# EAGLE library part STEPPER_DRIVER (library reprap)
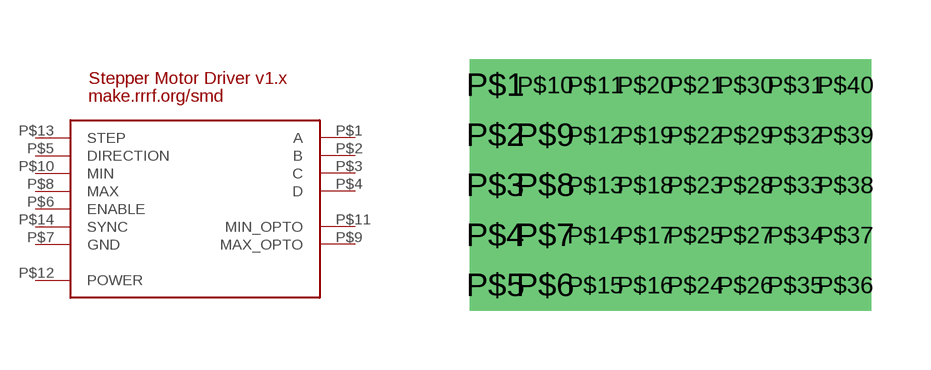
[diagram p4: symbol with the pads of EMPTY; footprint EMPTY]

Designator prefix -

## STEPPER_DRIVER  [EMPTY]
P$1  A
P$2  B
P$3  C
P$4  D
P$5  DIRECTION
P$6  ENABLE
P$7  GND
P$8  MAX
P$9  MAX_OPTO
P$10  MIN
P$11  MIN_OPTO
P$12  POWER
P$13  STEP
P$14  SYNC

## Footprint EMPTY (pad centres in mm)
drill 0.8 square: P$1 -1.27,5.08; P$2 -1.27,3.81; P$3 -1.27,2.54; P$4 -1.27,1.27; P$5 -1.27,0; P$6 0,0; P$7 0,1.27; P$8 0,2.54; P$9 0,3.81; P$10 0,5.08; P$11 1.27,5.08; P$12 1.27,3.81; P$13 1.27,2.54; P$14 1.27,1.27; P$15 1.27,0; P$16 2.54,0; P$17 2.54,1.27; P$18 2.54,2.54; P$19 2.54,3.81; P$20 2.54,5.08; P$21 3.81,5.08; P$22 3.81,3.81; P$23 3.81,2.54; P$24 3.81,0; P$25 3.81,1.27; P$26 5.08,0; P$27 5.08,1.27; P$28 5.08,2.54; P$29 5.08,3.81; P$30 5.08,5.08; P$31 6.35,5.08; P$32 6.35,3.81; P$33 6.35,2.54; P$34 6.35,1.27; P$35 6.35,0; P$36 7.62,0; P$37 7.62,1.27; P$38 7.62,2.54; P$39 7.62,3.81; P$40 7.62,5.08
